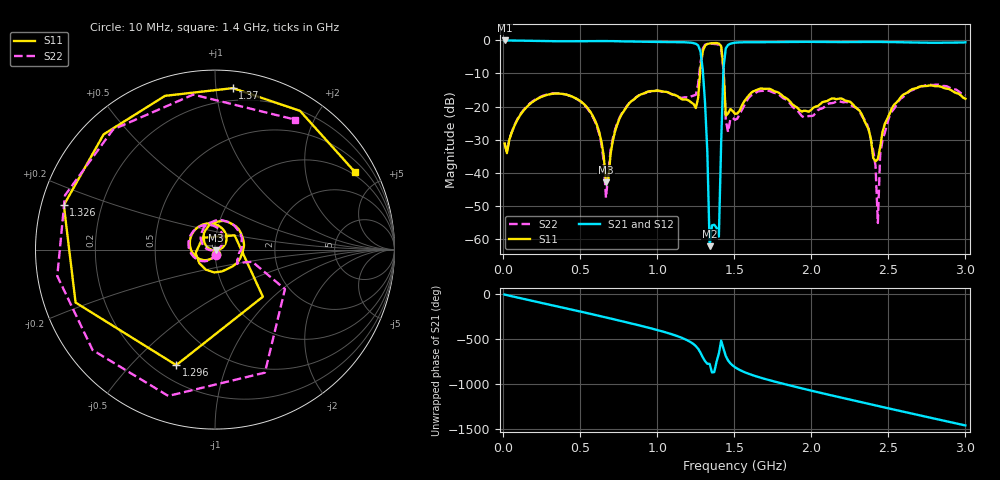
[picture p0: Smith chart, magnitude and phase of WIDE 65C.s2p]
!Agilent Technologies,E8363B,SG43030131,A.07.50.48
!Agilent E8363B: A.07.50.48
!Date: Friday, November 21, 2025 21:35:20
!Correction: S11(Full 2 Port(1,2))
!S21(Full 2 Port(1,2))
!S12(Full 2 Port(1,2))
!S22(Full 2 Port(1,2))
!S2P File: Measurements: S11, S21, S12, S22:
# Hz S  dB  R 50
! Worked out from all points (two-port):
!   201 points, 10 MHz to 3 GHz, reference 50 ohm
!   highest |S21| = -0.07 dB at 10 MHz (marker M1); lowest = -62.1 dB at 1.341 GHz (marker M2)
!   |S21| within 3 dB of the highest: start of sweep to 1.279 GHz; 1.444 GHz to end of sweep
!   lowest |S11| = -42.9 dB at 667.8 MHz (marker M3), VSWR 1.01, Z = 50.6 - j0.409 ohm
!   |S11| at or under -10 dB: start of sweep to 1.278 GHz; 1.432 GHz to end of sweep
!   |S22| runs from -55.1 to -1.0 dB; largest |S21 - S12| = 0.0028
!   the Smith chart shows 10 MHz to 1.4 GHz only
!   S11 on the Smith chart (normalised r, x): 10 MHz: 1.01, -0.05; 1.296 GHz: 0.28, -0.68; 1.326 GHz: 0.07, +0.14; 1.37 GHz: 0.11, +1.11; 1.4 GHz: 0.87, +3.65
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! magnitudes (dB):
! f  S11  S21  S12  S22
! 10 MHz  -31.1  -0.1  0.0  -31.1
! 518.3 MHz  -19.0  -0.3  -0.3  -19.1
! 623 MHz  -27.6  -0.3  -0.2  -28.1
! 667.8 MHz  -42.9  -0.3  -0.3  -47.5
! 757.5 MHz  -23.4  -0.3  -0.3  -23.2
! 1.012 GHz  -15.2  -0.5  -0.5  -15.3
! 1.251 GHz  -20.4  -1.1  -1.1  -16.5
! 1.296 GHz  -3.4  -8.8  -8.9  -2.6
! 1.326 GHz  -1.1  -33.8  -33.9  -1.1
! 1.341 GHz  -1.0  -62.1  -62.3  -1.0
! 1.37 GHz  -0.9  -55.6  -55.8  -1.1
! 1.4 GHz  -1.0  -59.2  -59.1  -1.4
! 1.43 GHz  -8.4  -8.4  -8.4  -9.0
! 1.46 GHz  -22.0  -1.4  -1.4  -27.7
! 1.505 GHz  -22.2  -0.8  -0.8  -24.0
! 2.013 GHz  -20.3  -0.5  -0.5  -22.7
! 2.357 GHz  -25.4  -0.5  -0.5  -24.7
! 2.417 GHz  -36.5  -0.5  -0.5  -37.9
! 2.432 GHz  -35.9  -0.5  -0.5  -55.1
! 2.447 GHz  -32.2  -0.5  -0.5  -34.6
! 2.507 GHz  -22.3  -0.5  -0.5  -23.0
! 3 GHz  -17.6  -0.6  -0.6  -16.6
